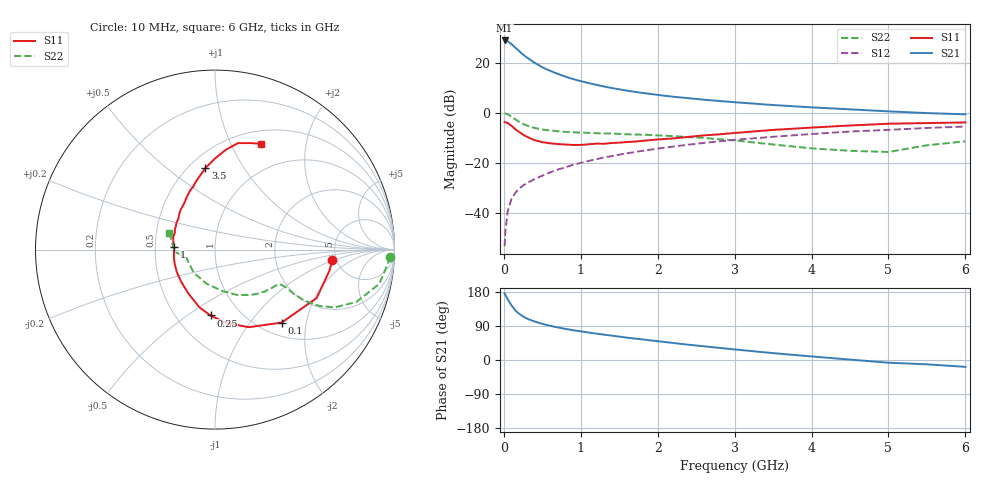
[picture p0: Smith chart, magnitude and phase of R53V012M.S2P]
! SIEMENS Small Signal Semiconductors
! BFR183
! Si NPN RF Bipolar Junction Transistor in SOT23
! VCE = 3 V  IC = 12 mA
! Common Emitter S-Parameters:  May  1996
# GHz  S  MA  R  50
!  f  S11  S21  S12  S22
! GHz  MAG  ANG  MAG  ANG  MAG  ANG  MAG  ANG
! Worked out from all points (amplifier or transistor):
!   36 points, 10 MHz to 6 GHz, reference 50 ohm
!   highest |S21| = 28.9 dB at 10 MHz (marker M1)
!   |S21| within 3 dB of that: start of sweep to 155 MHz
!   unconditionally stable (mu >= 1): 726.7 MHz to 2.442 GHz
!   at 250 MHz: K = 0.67, MSG = 26.1 dB, |S12| = -28.9 dB
!   at 1.4 GHz: K = 1.05, MAG = 12.2 dB, |S12| = -17.3 dB
!   at 6 GHz: K = 0.90, MSG = 2.4 dB, |S12| = -5.4 dB
!   S11 on the Smith chart (normalised r, x): 10 MHz: 4.62, -0.97; 100 MHz: 1.24, -1.45; 250 MHz: 0.73, -0.62; 1 GHz: 0.63, +0.02; 3.5 GHz: 0.60, +0.69; 6 GHz: 0.65, +1.31
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0.01  0.6572 -5.2  27.73 175.9  0.0022 91.5  0.9773 -2.4
0.02  0.6482 -10.5  27.73 171.6  0.0043 81.6  0.9652 -4.8
0.05  0.6274 -25.5  26.77 160.3  0.0108 78.1  0.935 -11.8
0.1  0.5507 -47.6  23.45 144.0  0.0193 72.5  0.8387 -20.4
0.15  0.4713 -66.5  19.95 130.8  0.0255 66.2  0.7407 -25.8
0.2  0.4146 -81.1  16.96 121.8  0.0308 64.7  0.663 -28.3
0.25  0.3679 -93.9  14.5 114.8  0.0357 63.8  0.6025 -29.3
0.3  0.3337 -104.9  12.63 109.2  0.0397 64.0  0.5595 -29.7
0.4  0.2849 -121.9  9.955 101.6  0.0479 65.0  0.5001 -29.2
0.5  0.2604 -136.1  8.112 95.3  0.0559 66.0  0.465 -28.4
0.6  0.2474 -148.9  6.897 90.3  0.0649 66.7  0.4449 -28.0
0.7  0.2387 -159.5  5.992 86.0  0.0739 67.3  0.4303 -28.0
0.8  0.2339 -168.1  5.269 82.1  0.0823 67.1  0.4181 -28.0
1  0.2294 175.8  4.277 75.6  0.1007 67.1  0.4043 -28.8
1.1  0.2355 170.2  3.931 72.6  0.1099 66.7  0.3988 -29.9
1.3  0.2416 158.2  3.353 67.0  0.1285 65.6  0.3886 -31.7
1.6  0.262 144.9  2.769 59.0  0.1562 63.6  0.3738 -35.6
2.2  0.3086 123.9  2.097 45.0  0.2127 58.3  0.3442 -45.4
3.5  0.4571 96.7  1.432 18.1  0.3337 43.0  0.2337 -80.1
4.5  0.5596 83.8  1.175 1.1  0.4242 30.6  0.1753 -132.6
5.5  0.6258 71.5  0.989 -11.4  0.4995 18.6  0.2256 -177.3
6  0.6434 66.3  0.934 -18.1  0.5343 11.0  0.2707 160.0
